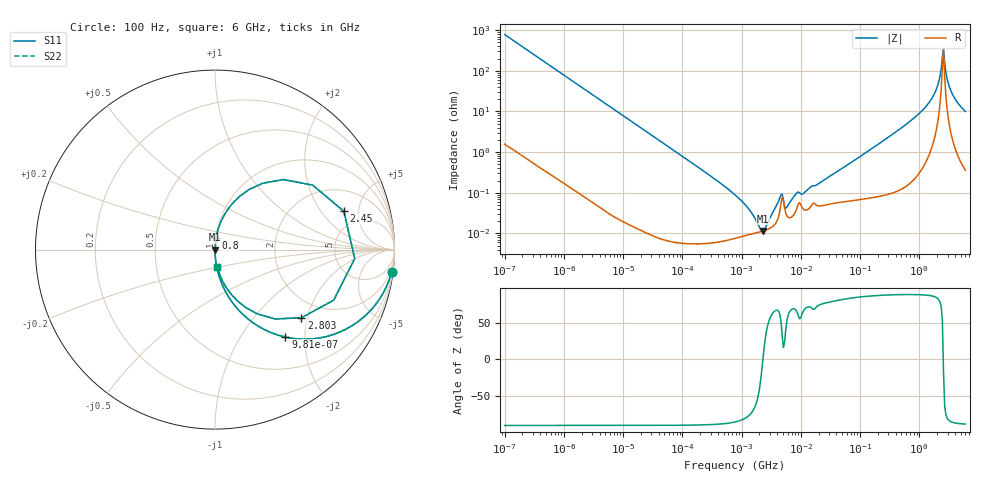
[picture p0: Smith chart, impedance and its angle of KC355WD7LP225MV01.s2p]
!Murata Part Number: KC355WD7LP225MV01
!These Parameters are Measured in Series Mode Connection
!Data Generated on Jun 19, 2026
!  o--ll--o
!Port1  Port2
!  o------o
!Operation Temp=25[degC], DC Bias Voltage=0[V]
!Freq. Start=100[Hz] Stop=6[GHz] 401[Steps]
# Hz S RI R 50
!Freq.(Hz) S11(Real) S11(Imag) S21(Real) S21(Imag) S12(Real) S12(Imag) S22(Real) S22(Imag)
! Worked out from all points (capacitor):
!   401 points, 100 Hz to 6 GHz, reference 50 ohm
!   read as one part in series: C = 2.02 uF near 109 Hz
!   lowest |Z| = 11.4 mohm at 2.269 MHz (marker M1)
!   series resonance near 2.29 MHz, so ESL is about 2.4 nH
!   S11 on the Smith chart (normalised r, x): 100 Hz: 1, -16; 981 Hz: 1.00, -1.61; 800 MHz: 1.00, +0.14; 2.45 GHz: 3.50, +3.41; 2.803 GHz: 1.51, -1.84; 6 GHz: 1.01, -0.20
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100  0.9838 -0.1252  0.0162 0.1252  0.0162 0.1252  0.9838 -0.1252
335  0.846 -0.3599  0.154 0.3599  0.154 0.3599  0.846 -0.3599
981  0.3923 -0.4872  0.6077 0.4872  0.6077 0.4872  0.3923 -0.4872
2008  0.1342 -0.3397  0.8658 0.3397  0.8658 0.3397  0.1342 -0.3397
7036  0.0127 -0.1108  0.9873 0.1108  0.9873 0.1108  0.0127 -0.1108
40335  0.000461 -0.0196  0.9995 0.0196  0.9995 0.0196  0.000461 -0.0196
774597  7.63e-05 -0.000889  0.9999 0.000889  0.9999 0.000889  7.63e-05 -0.000889
1325623  9.3e-05 -0.000387  0.9999 0.000387  0.9999 0.000387  9.3e-05 -0.000387
2268635  0.000114 -6.4e-06  0.9999 6.4e-06  0.9999 6.4e-06  0.000114 -6.4e-06
4440638  0.000369 0.000666  0.9996 -0.000666  0.9996 -0.000666  0.000369 0.000666
5809218  0.000272 0.000349  0.9997 -0.000349  0.9997 -0.000349  0.000272 0.000349
8311524  0.000367 0.000865  0.9996 -0.000865  0.9996 -0.000865  0.000367 0.000865
1.555665e7  0.000523 0.00137  0.9995 -0.00137  0.9995 -0.00137  0.000523 0.00137
3.124326e8  0.00152 0.0242  0.9985 -0.0242  0.9985 -0.0242  0.00152 0.0242
8.000355e8  0.00658 0.067  0.9934 -0.067  0.9934 -0.067  0.00658 0.067
1.791126e9  0.0842 0.2412  0.9158 -0.2412  0.9158 -0.2412  0.0842 0.2412
2.142435e9  0.2667 0.37  0.7333 -0.37  0.7333 -0.37  0.2667 0.37
2.450438e9  0.7178 0.2139  0.2822 -0.2139  0.2822 -0.2139  0.7178 0.2139
2.802721e9  0.4817 -0.3797  0.5183 0.3797  0.5183 0.3797  0.4817 -0.3797
3.065283e9  0.2363 -0.3584  0.7637 0.3584  0.7637 0.3584  0.2363 -0.3584
3.505958e9  0.0985 -0.2583  0.9015 0.2583  0.9015 0.2583  0.0985 -0.2583
6e9  0.0133 -0.0981  0.9867 0.0981  0.9867 0.0981  0.0133 -0.0981
